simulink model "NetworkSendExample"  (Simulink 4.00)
settings: Solver=FixedStepDiscrete  StartTime=0.0  StopTime=100000.0  FixedStep=0.02  RelTol=1e-3
libraries: AVDSBlockset x4, simulink3 x1

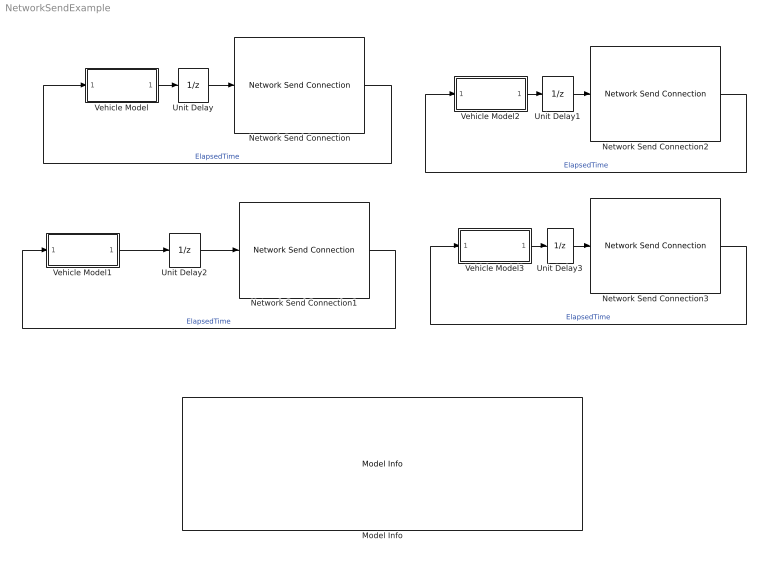
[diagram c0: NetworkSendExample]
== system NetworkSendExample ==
  Model Info : simulink3/Signals & Systems/Model Info  InitialBlockCM=none  BlockCM=none  Frame=on  DisplayStringWithTags=|  HorizontalTextAlignment=Left  LeftAlignmentValue=0.02  SourceBlockDiagram=NetworkSendExample  TagMaxNumber=20
      | NetworkSendExample.mdl - Simulink example that sends vehicle packets out on the 
      |    local network.
      |    - Run AVDS
      |    - In AVDS, select "Network" and "Observer" modes. 
      |    - Open the NetworkSendExample model file.
      |    - Start the Simulink simulation.
      |    - In AVDS, select the vehicle to view from AVDS's "Aircraft Image" menu:
      |      select "Initialize->Aircraft Image"
      |    - Press the AVDS Start button.
  Network Send Connection : AVDSBlockset/Network Send Connection  Description=This block is used to connect Simulink to AVDS through the MATLAB AC model.  VehicleHandleName=SimulinkVehicle01  TransmitRateHz=30  CraftType=1  InitLatitudeDeg=37.981523  InitLongitudeDeg=-122.063400  InitAltitudeFeet=10000  RealTime=on
  Network Send Connection1 : AVDSBlockset/Network Send Connection  Description=This block is used to connect Simulink to AVDS through the MATLAB AC model.  VehicleHandleName=SimulinkVehicle01  TransmitRateHz=30  CraftType=2  InitLatitudeDeg=37.981523  InitLongitudeDeg=-122.063400  InitAltitudeFeet=10000  RealTime=on
  Network Send Connection2 : AVDSBlockset/Network Send Connection  Description=This block is used to connect Simulink to AVDS through the MATLAB AC model.  VehicleHandleName=SimulinkVehicle01  TransmitRateHz=30  CraftType=3  InitLatitudeDeg=37.981523  InitLongitudeDeg=-122.063400  InitAltitudeFeet=10000  RealTime=on
  Network Send Connection3 : AVDSBlockset/Network Send Connection  Description=This block is used to connect Simulink to AVDS through the MATLAB AC model.  VehicleHandleName=SimulinkVehicle01  TransmitRateHz=30  CraftType=4  InitLatitudeDeg=37.981523  InitLongitudeDeg=-122.063400  InitAltitudeFeet=10000  RealTime=on
  Unit Delay{,1..3} (4 alike) : UnitDelay  X0=0  SampleTime=0.02
  Vehicle Model : Subsystem
  Vehicle Model1 : Subsystem
  Vehicle Model2 : Subsystem
  Vehicle Model3 : Subsystem
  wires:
  Vehicle Model/1(Out1) -> Unit Delay/1
  Network Send Connection/1 -> Vehicle Model/1(In1)  "ElapsedTime"
  Network Send Connection1/1 -> Vehicle Model1/1(In1)  "ElapsedTime"
  Vehicle Model2/1(Out1) -> Unit Delay1/1
  Network Send Connection2/1 -> Vehicle Model2/1(In1)  "ElapsedTime"
  Vehicle Model3/1(Out1) -> Unit Delay3/1
  Network Send Connection3/1 -> Vehicle Model3/1(In1)  "ElapsedTime"
  Unit Delay/1 -> Network Send Connection/1
  Vehicle Model1/1(Out1) -> Unit Delay2/1
  Unit Delay2/1 -> Network Send Connection1/1
  Unit Delay1/1 -> Network Send Connection2/1
  Unit Delay3/1 -> Network Send Connection3/1

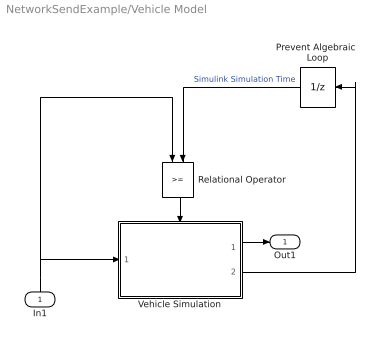
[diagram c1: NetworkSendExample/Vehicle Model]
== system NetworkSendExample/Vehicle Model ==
  In1 : Inport  Orientation=up  Port=1  LatchInput=off
  Prevent Algebraic  Loop : UnitDelay  Orientation=left  X0=0  SampleTime=0.02
  Relational Operator : RelationalOperator  Orientation=down  Operator=>=
  Vehicle Simulation : Subsystem  TreatAsAtomicUnit=on
  Out1 : Outport  Port=1
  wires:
  Relational Operator/1 -> Vehicle Simulation/Enable
  Vehicle Simulation/2(Vehicle Simulation  Time) -> Prevent Algebraic  Loop/1
  Prevent Algebraic  Loop/1 -> Relational Operator/2  "Simulink Simulation Time"
  In1/1 -> Vehicle Simulation/1(In1), Relational Operator/1
  Vehicle Simulation/1(Out To  AVDS Network) -> Out1/1

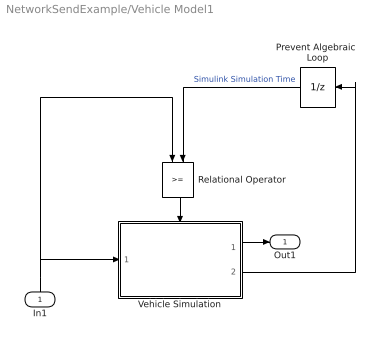
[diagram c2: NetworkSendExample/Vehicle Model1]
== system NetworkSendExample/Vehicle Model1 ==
  In1 : Inport  Orientation=up  Port=1  LatchInput=off
  Prevent Algebraic  Loop : UnitDelay  Orientation=left  X0=0  SampleTime=0.02
  Relational Operator : RelationalOperator  Orientation=down  Operator=>=
  Vehicle Simulation : Subsystem  TreatAsAtomicUnit=on
  Out1 : Outport  Port=1
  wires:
  Vehicle Simulation/1(Out To  AVDS Network) -> Out1/1
  In1/1 -> Relational Operator/1, Vehicle Simulation/1(In1)
  Prevent Algebraic  Loop/1 -> Relational Operator/2  "Simulink Simulation Time"
  Vehicle Simulation/2(Vehicle Simulation  Time) -> Prevent Algebraic  Loop/1
  Relational Operator/1 -> Vehicle Simulation/Enable

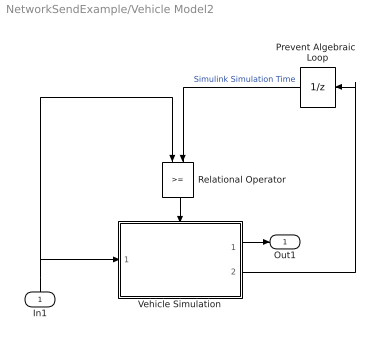
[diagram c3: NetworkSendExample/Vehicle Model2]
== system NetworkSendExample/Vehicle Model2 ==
  In1 : Inport  Orientation=up  Port=1  LatchInput=off
  Prevent Algebraic  Loop : UnitDelay  Orientation=left  X0=0  SampleTime=0.02
  Relational Operator : RelationalOperator  Orientation=down  Operator=>=
  Vehicle Simulation : Subsystem  TreatAsAtomicUnit=on
  Out1 : Outport  Port=1
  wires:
  Relational Operator/1 -> Vehicle Simulation/Enable
  Vehicle Simulation/2(Vehicle Simulation  Time) -> Prevent Algebraic  Loop/1
  Prevent Algebraic  Loop/1 -> Relational Operator/2  "Simulink Simulation Time"
  In1/1 -> Vehicle Simulation/1(In1), Relational Operator/1
  Vehicle Simulation/1(Out To  AVDS Network) -> Out1/1

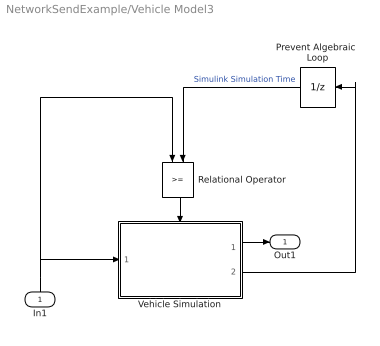
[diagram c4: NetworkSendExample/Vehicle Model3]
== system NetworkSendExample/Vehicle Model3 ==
  In1 : Inport  Orientation=up  Port=1  LatchInput=off
  Prevent Algebraic  Loop : UnitDelay  Orientation=left  X0=0  SampleTime=0.02
  Relational Operator : RelationalOperator  Orientation=down  Operator=>=
  Vehicle Simulation : Subsystem  TreatAsAtomicUnit=on
  Out1 : Outport  Port=1
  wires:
  Vehicle Simulation/1(Out To  AVDS Network) -> Out1/1
  In1/1 -> Relational Operator/1, Vehicle Simulation/1(In1)
  Prevent Algebraic  Loop/1 -> Relational Operator/2  "Simulink Simulation Time"
  Vehicle Simulation/2(Vehicle Simulation  Time) -> Prevent Algebraic  Loop/1
  Relational Operator/1 -> Vehicle Simulation/Enable

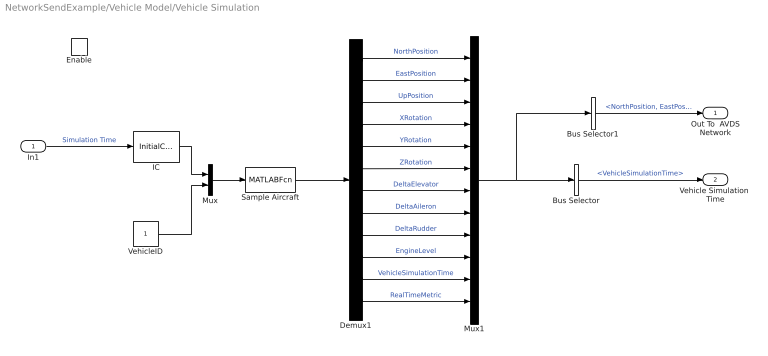
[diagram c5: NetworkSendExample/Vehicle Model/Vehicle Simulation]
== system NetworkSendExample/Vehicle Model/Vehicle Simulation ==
  In1 : Inport  Port=1  LatchInput=off
  Enable : EnablePort
  Bus Selector : BusSelector  OutputSignals=VehicleSimulationTime  MuxedOutput=off
  Bus Selector1 : BusSelector  OutputSignals=NorthPosition,EastPosition,UpPosition,XRotation,YRotation,ZRotation,DeltaElevator,DeltaAileron,DeltaRudder,EngineLevel  MuxedOutput=on
  Demux1 : Demux  Outputs=12  BusSelectionMode=off
  IC : InitialCondition  Value=0
  Mux : Mux  Inputs=2
  Mux1 : Mux  Inputs=12
  Sample Aircraft : MATLABFcn  MATLABFcn=NetworkSendSimulink  OutputDimensions=12  OutputSignalType=auto  Output1D=on
  VehicleID : Constant  Value=1
  Out To  AVDS Network : Outport  Port=1
  Vehicle Simulation  Time : Outport  Port=2
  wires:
  Bus Selector/1 -> Vehicle Simulation  Time/1  "<VehicleSimulationTime>"
  Demux1/1 -> Mux1/1  "NorthPosition"
  Demux1/2 -> Mux1/2  "EastPosition"
  Demux1/3 -> Mux1/3  "UpPosition"
  Demux1/4 -> Mux1/4  "XRotation"
  Demux1/5 -> Mux1/5  "YRotation"
  Demux1/6 -> Mux1/6  "ZRotation"
  Demux1/7 -> Mux1/7  "DeltaElevator"
  Demux1/8 -> Mux1/8  "DeltaAileron"
  Demux1/9 -> Mux1/9  "DeltaRudder"
  Demux1/10 -> Mux1/10  "EngineLevel"
  Sample Aircraft/1 -> Demux1/1
  Mux1/1 -> Bus Selector/1, Bus Selector1/1
  Bus Selector1/1 -> Out To  AVDS Network/1  "<NorthPosition, EastPosition, UpPosition, XRotation, YRotation, ZRotation, DeltaElevator, DeltaAileron, DeltaRudder, EngineLevel>"
  Demux1/11 -> Mux1/11  "VehicleSimulationTime"
  Demux1/12 -> Mux1/12  "RealTimeMetric"
  Mux/1 -> Sample Aircraft/1
  In1/1 -> IC/1  "Simulation Time"
  IC/1 -> Mux/1
  VehicleID/1 -> Mux/2

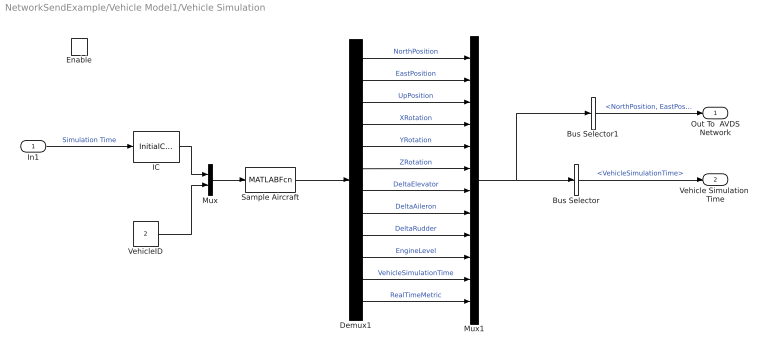
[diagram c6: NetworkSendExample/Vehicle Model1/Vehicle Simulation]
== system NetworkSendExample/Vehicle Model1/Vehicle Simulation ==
  In1 : Inport  Port=1  LatchInput=off
  Enable : EnablePort
  Bus Selector : BusSelector  OutputSignals=VehicleSimulationTime  MuxedOutput=off
  Bus Selector1 : BusSelector  OutputSignals=NorthPosition,EastPosition,UpPosition,XRotation,YRotation,ZRotation,DeltaElevator,DeltaAileron,DeltaRudder,EngineLevel  MuxedOutput=on
  Demux1 : Demux  Outputs=12  BusSelectionMode=off
  IC : InitialCondition  Value=0
  Mux : Mux  Inputs=2
  Mux1 : Mux  Inputs=12
  Sample Aircraft : MATLABFcn  MATLABFcn=NetworkSendSimulink  OutputDimensions=12  OutputSignalType=auto  Output1D=on
  VehicleID : Constant  Value=2
  Out To  AVDS Network : Outport  Port=1
  Vehicle Simulation  Time : Outport  Port=2
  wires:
  VehicleID/1 -> Mux/2
  IC/1 -> Mux/1
  In1/1 -> IC/1  "Simulation Time"
  Mux/1 -> Sample Aircraft/1
  Demux1/12 -> Mux1/12  "RealTimeMetric"
  Demux1/11 -> Mux1/11  "VehicleSimulationTime"
  Bus Selector1/1 -> Out To  AVDS Network/1  "<NorthPosition, EastPosition, UpPosition, XRotation, YRotation, ZRotation, DeltaElevator, DeltaAileron, DeltaRudder, EngineLevel>"
  Mux1/1 -> Bus Selector1/1, Bus Selector/1
  Sample Aircraft/1 -> Demux1/1
  Demux1/10 -> Mux1/10  "EngineLevel"
  Demux1/9 -> Mux1/9  "DeltaRudder"
  Demux1/8 -> Mux1/8  "DeltaAileron"
  Demux1/7 -> Mux1/7  "DeltaElevator"
  Demux1/6 -> Mux1/6  "ZRotation"
  Demux1/5 -> Mux1/5  "YRotation"
  Demux1/4 -> Mux1/4  "XRotation"
  Demux1/3 -> Mux1/3  "UpPosition"
  Demux1/2 -> Mux1/2  "EastPosition"
  Demux1/1 -> Mux1/1  "NorthPosition"
  Bus Selector/1 -> Vehicle Simulation  Time/1  "<VehicleSimulationTime>"

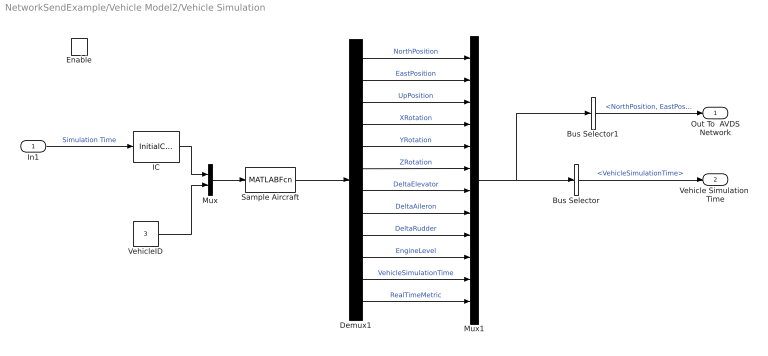
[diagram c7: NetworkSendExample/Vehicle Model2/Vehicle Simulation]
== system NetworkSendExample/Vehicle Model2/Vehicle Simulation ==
  In1 : Inport  Port=1  LatchInput=off
  Enable : EnablePort
  Bus Selector : BusSelector  OutputSignals=VehicleSimulationTime  MuxedOutput=off
  Bus Selector1 : BusSelector  OutputSignals=NorthPosition,EastPosition,UpPosition,XRotation,YRotation,ZRotation,DeltaElevator,DeltaAileron,DeltaRudder,EngineLevel  MuxedOutput=on
  Demux1 : Demux  Outputs=12  BusSelectionMode=off
  IC : InitialCondition  Value=0
  Mux : Mux  Inputs=2
  Mux1 : Mux  Inputs=12
  Sample Aircraft : MATLABFcn  MATLABFcn=NetworkSendSimulink  OutputDimensions=12  OutputSignalType=auto  Output1D=on
  VehicleID : Constant  Value=3
  Out To  AVDS Network : Outport  Port=1
  Vehicle Simulation  Time : Outport  Port=2
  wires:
  Bus Selector/1 -> Vehicle Simulation  Time/1  "<VehicleSimulationTime>"
  Demux1/1 -> Mux1/1  "NorthPosition"
  Demux1/2 -> Mux1/2  "EastPosition"
  Demux1/3 -> Mux1/3  "UpPosition"
  Demux1/4 -> Mux1/4  "XRotation"
  Demux1/5 -> Mux1/5  "YRotation"
  Demux1/6 -> Mux1/6  "ZRotation"
  Demux1/7 -> Mux1/7  "DeltaElevator"
  Demux1/8 -> Mux1/8  "DeltaAileron"
  Demux1/9 -> Mux1/9  "DeltaRudder"
  Demux1/10 -> Mux1/10  "EngineLevel"
  Sample Aircraft/1 -> Demux1/1
  Mux1/1 -> Bus Selector/1, Bus Selector1/1
  Bus Selector1/1 -> Out To  AVDS Network/1  "<NorthPosition, EastPosition, UpPosition, XRotation, YRotation, ZRotation, DeltaElevator, DeltaAileron, DeltaRudder, EngineLevel>"
  Demux1/11 -> Mux1/11  "VehicleSimulationTime"
  Demux1/12 -> Mux1/12  "RealTimeMetric"
  Mux/1 -> Sample Aircraft/1
  In1/1 -> IC/1  "Simulation Time"
  IC/1 -> Mux/1
  VehicleID/1 -> Mux/2

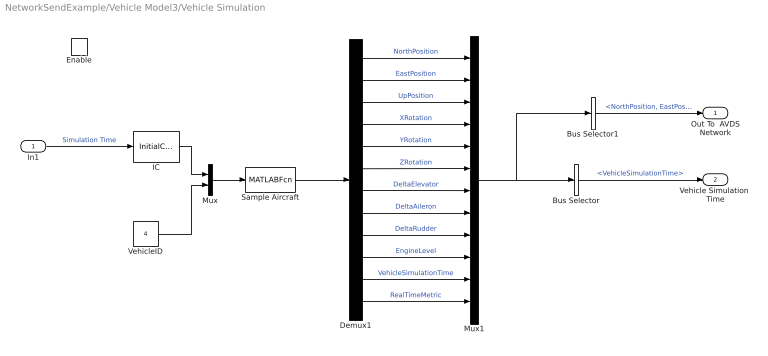
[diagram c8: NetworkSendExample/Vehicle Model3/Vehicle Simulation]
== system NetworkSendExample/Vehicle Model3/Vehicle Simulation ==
  In1 : Inport  Port=1  LatchInput=off
  Enable : EnablePort
  Bus Selector : BusSelector  OutputSignals=VehicleSimulationTime  MuxedOutput=off
  Bus Selector1 : BusSelector  OutputSignals=NorthPosition,EastPosition,UpPosition,XRotation,YRotation,ZRotation,DeltaElevator,DeltaAileron,DeltaRudder,EngineLevel  MuxedOutput=on
  Demux1 : Demux  Outputs=12  BusSelectionMode=off
  IC : InitialCondition  Value=0
  Mux : Mux  Inputs=2
  Mux1 : Mux  Inputs=12
  Sample Aircraft : MATLABFcn  MATLABFcn=NetworkSendSimulink  OutputDimensions=12  OutputSignalType=auto  Output1D=on
  VehicleID : Constant  Value=4
  Out To  AVDS Network : Outport  Port=1
  Vehicle Simulation  Time : Outport  Port=2
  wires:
  VehicleID/1 -> Mux/2
  IC/1 -> Mux/1
  In1/1 -> IC/1  "Simulation Time"
  Mux/1 -> Sample Aircraft/1
  Demux1/12 -> Mux1/12  "RealTimeMetric"
  Demux1/11 -> Mux1/11  "VehicleSimulationTime"
  Bus Selector1/1 -> Out To  AVDS Network/1  "<NorthPosition, EastPosition, UpPosition, XRotation, YRotation, ZRotation, DeltaElevator, DeltaAileron, DeltaRudder, EngineLevel>"
  Mux1/1 -> Bus Selector1/1, Bus Selector/1
  Sample Aircraft/1 -> Demux1/1
  Demux1/10 -> Mux1/10  "EngineLevel"
  Demux1/9 -> Mux1/9  "DeltaRudder"
  Demux1/8 -> Mux1/8  "DeltaAileron"
  Demux1/7 -> Mux1/7  "DeltaElevator"
  Demux1/6 -> Mux1/6  "ZRotation"
  Demux1/5 -> Mux1/5  "YRotation"
  Demux1/4 -> Mux1/4  "XRotation"
  Demux1/3 -> Mux1/3  "UpPosition"
  Demux1/2 -> Mux1/2  "EastPosition"
  Demux1/1 -> Mux1/1  "NorthPosition"
  Bus Selector/1 -> Vehicle Simulation  Time/1  "<VehicleSimulationTime>"
